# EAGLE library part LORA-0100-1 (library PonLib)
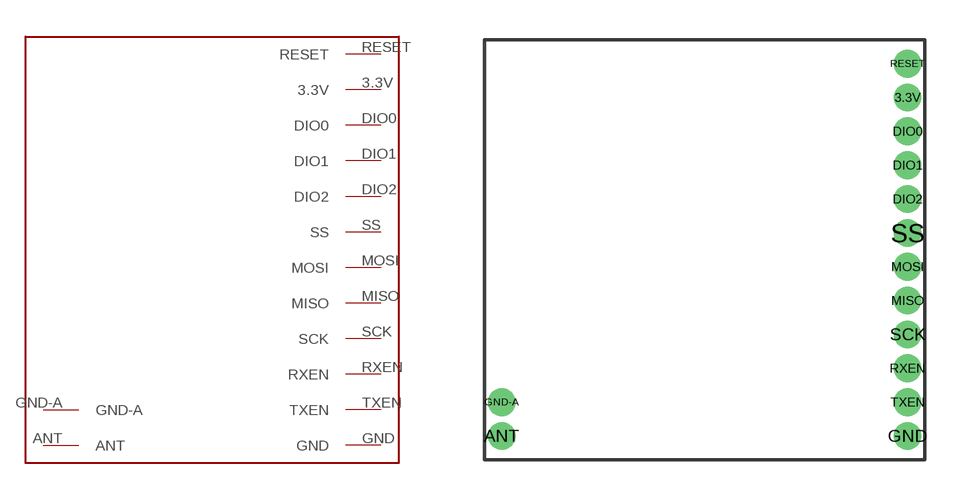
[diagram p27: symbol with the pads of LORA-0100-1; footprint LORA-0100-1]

Designator prefix -

## LORA-0100-1  [LORA-0100-1]
3.3V  3.3V
ANT  ANT
DIO0  DIO0
DIO1  DIO1
DIO2  DIO2
GND  GND
GND-A  GND-A
MISO  MISO
MOSI  MOSI
RESET  RESET
RXEN  RXEN
SCK  SCK
SS  SS
TXEN  TXEN

## Footprint LORA-0100-1 (pad centres in mm)
drill 0.533 pad 0.889: 3.3V 7.62,5.715; ANT -7.62,-6.985; DIO0 7.62,4.445; DIO1 7.62,3.175; DIO2 7.62,1.905; GND 7.62,-6.985; GND-A -7.62,-5.715; MISO 7.62,-1.905; MOSI 7.62,-0.635; RESET 7.62,6.985; RXEN 7.62,-4.445; SCK 7.62,-3.175; SS 7.62,0.635; TXEN 7.62,-5.715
